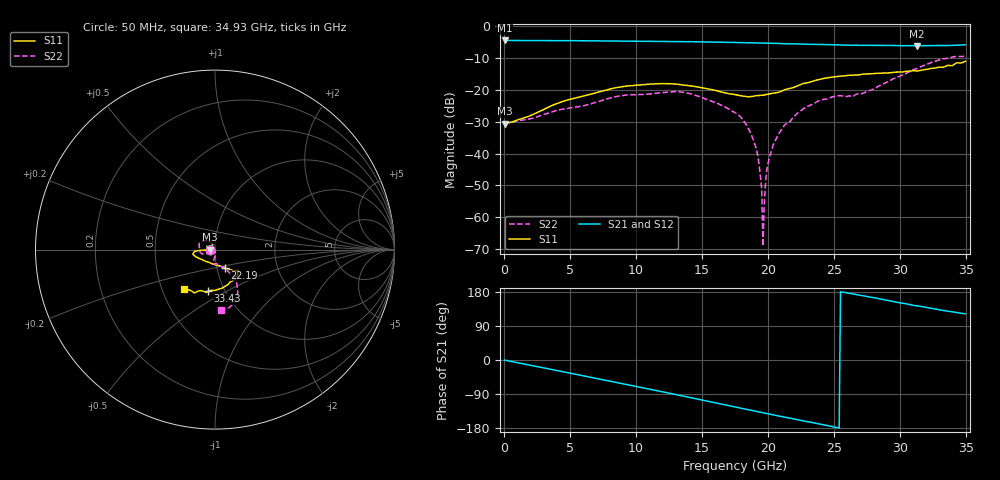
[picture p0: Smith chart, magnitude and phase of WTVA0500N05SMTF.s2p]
! 50 ohm 2-Port S-parameters measured by Modelithics Inc support@modelithics.com  Tampa, FL USA 813-866-6335 (February 2024)
! Smiths Interconnect,  5dB P/N: WTVA0500N05SMTF, Temperature: 50 C
! Board: 10 mil Rogers 4350B, Mounting Pad Dimensions: Length: 15 mils, Width: 25 mils, Gap: 40 mils.
# Hz S RI R 50
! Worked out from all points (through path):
!   352 points, 50 MHz to 34.93 GHz, reference 50 ohm
!   highest |S21| = -4.45 dB at 50 MHz (marker M1); lowest = -6.1 dB at 31.24 GHz (marker M2)
!   group delay of S21, straight-line fit = 19.3 ps
!   lowest |S11| = -30.6 dB at 50 MHz (marker M3), VSWR 1.06, Z = 47.1 + j0.0138 ohm
!   |S11| at or under -10 dB: start of sweep to end of sweep
!   |S22| runs from -69.1 to -9.4 dB; largest |S21 - S12| = 0.0063
!   S11 on the Smith chart (normalised r, x): 50 MHz: 0.94, +0.00; 22.19 GHz: 1.10, -0.22; 33.43 GHz: 0.83, -0.41; 34.93 GHz: 0.64, -0.31
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5e7  -0.0294 0.000146  0.599 -0.00329  0.5985 -0.00324  -0.0289 -0.0017
5.8715e9  -0.0788 -0.00385  0.4483 -0.3876  0.4479 -0.3873  -0.05 -0.0241
8.757e9  -0.1106 -0.00875  0.2839 -0.513  0.2828 -0.5129  -0.0783 -0.0192
1.1742e10  -0.1233 -0.0235  0.079 -0.5735  0.0777 -0.5731  -0.0884 0.0167
1.42295e10  -0.1085 -0.0381  -0.1014 -0.5634  -0.1025 -0.5627  -0.0715 0.0477
1.7513e10  -0.0545 -0.0644  -0.3122 -0.4626  -0.3122 -0.4618  -0.0231 0.0373
1.8508e10  -0.0289 -0.0727  -0.3638 -0.4144  -0.3641 -0.4136  -0.00944 0.0228
1.92045e10  -0.0127 -0.0806  -0.3957 -0.3778  -0.3951 -0.3778  -0.00234 0.00917
1.9503e10  -0.00588 -0.0824  -0.4083 -0.362  -0.4082 -0.3612  -0.000102 0.00288
1.96025e10  -0.00352 -0.0826  -0.4124 -0.3565  -0.4123 -0.3556  0.000101 0.000337
1.9702e10  -0.000992 -0.0834  -0.4163 -0.3507  -0.4162 -0.3499  3.86e-05 -0.0016
1.98015e10  0.00148 -0.0844  -0.4201 -0.3452  -0.42 -0.3447  6.4e-05 -0.00362
1.9901e10  0.00364 -0.0851  -0.4241 -0.3395  -0.4237 -0.3392  0.000525 -0.00565
2.01e10  0.00777 -0.0865  -0.4318 -0.3284  -0.4315 -0.3278  0.001 -0.00877
2.09955e10  0.0283 -0.0911  -0.4598 -0.2734  -0.4594 -0.273  0.000698 -0.0238
2.21895e10  0.0564 -0.1006  -0.4876 -0.2032  -0.4877 -0.2015  -0.00101 -0.0428
2.33835e10  0.0821 -0.1106  -0.5048 -0.1309  -0.5044 -0.1308  -0.00657 -0.0603
2.7065e10  0.1301 -0.1175  -0.4946 0.0858  -0.4938 0.0875  0.0194 -0.085
2.91545e10  0.1258 -0.1362  -0.4597 0.1997  -0.4572 0.2037  0.071 -0.1178
3.1244e10  0.0882 -0.1779  -0.3943 0.2959  -0.3921 0.2979  0.118 -0.1821
3.3433e10  -0.0389 -0.2319  -0.3176 0.3822  -0.3146 0.3839  0.0999 -0.2939
3.49255e10  -0.1746 -0.2213  -0.2701 0.434  -0.2695 0.4335  0.036 -0.3367
